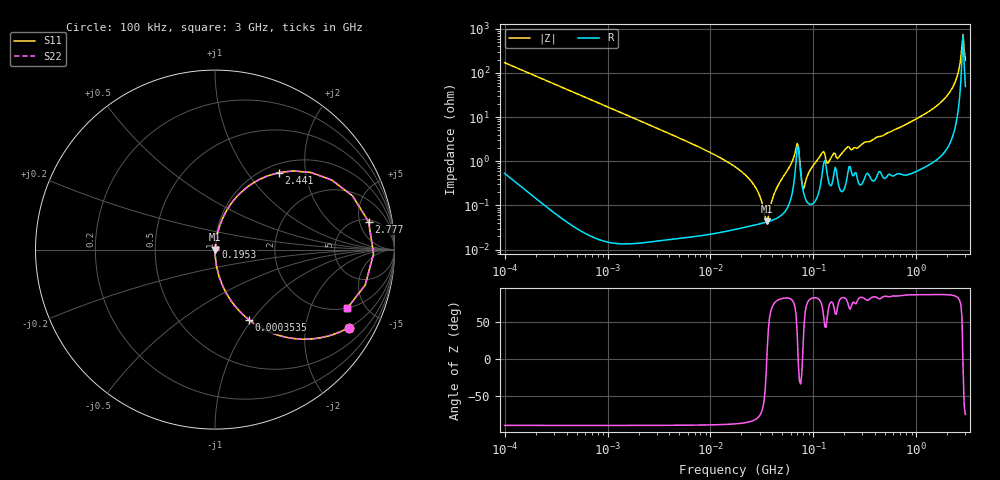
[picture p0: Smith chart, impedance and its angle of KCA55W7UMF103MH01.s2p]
!Murata Part Number: KCA55W7UMF103MH01
!These Parameters are Measured in Series Mode Connection
!Data Generated on Jan 08, 2026
!  o--ll--o
!Port1  Port2
!  o------o
!Operation Temp=25[degC], DC Bias Voltage=0[V]
!Freq. Start=100[kHz] Stop=3[GHz] 401[Steps]
# Hz S RI R 50
!Freq.(Hz) S11(Real) S11(Imag) S21(Real) S21(Imag) S12(Real) S12(Imag) S22(Real) S22(Imag)
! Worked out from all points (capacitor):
!   401 points, 100 kHz to 3 GHz, reference 50 ohm
!   read as one part in series: C = 9.31 nF near 105.3 kHz
!   lowest |Z| = 43.8 mohm at 35.64 MHz (marker M1)
!   series resonance near 35.29 MHz, so ESL is about 2.2 nH
!   S11 on the Smith chart (normalised r, x): 100 kHz: 1.01, -3.42; 353.5 kHz: 1.00, -0.97; 195.3 MHz: 1.00, +0.03; 2.441 GHz: 1.15, +1.43; 2.777 GHz: 5.40, +6.90; 3 GHz: 1.98, -3.71
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100000  0.7442 -0.4348  0.2558 0.4348  0.2558 0.4348  0.7442 -0.4348
353547  0.1898 -0.3916  0.8102 0.3916  0.8102 0.3916  0.1898 -0.3916
562235  0.0848 -0.2782  0.9152 0.2782  0.9152 0.2782  0.0848 -0.2782
3161081  0.00302 -0.0534  0.997 0.0534  0.997 0.0534  0.00302 -0.0534
1.77727e7  0.000342 -0.00722  0.9997 0.00722  0.9997 0.00722  0.000342 -0.00722
2.684345e7  0.000367 -0.00275  0.9996 0.00275  0.9996 0.00275  0.000367 -0.00275
3.564176e7  0.000425 0.000102  0.9996 -0.000102  0.9996 -0.000102  0.000425 0.000102
4.268829e7  0.0005 0.00206  0.9995 -0.00206  0.9995 -0.00206  0.0005 0.00206
6.788584e7  0.0101 0.0164  0.9899 -0.0164  0.9899 -0.0164  0.0101 0.0164
7.147675e7  0.0212 -0.00267  0.9788 0.00267  0.9788 0.00267  0.0212 -0.00267
7.722238e7  0.0032 -0.00119  0.9968 0.00119  0.9968 0.00119  0.0032 -0.00119
8.130716e7  0.00174 0.00187  0.9983 -0.00187  0.9983 -0.00187  0.00174 0.00187
9.738194e7  0.00113 0.00737  0.9989 -0.00737  0.9989 -0.00737  0.00113 0.00737
1.228043e8  0.00624 0.0147  0.9938 -0.0147  0.9938 -0.0147  0.00624 0.0147
1.39694e8  0.00374 0.0085  0.9963 -0.0085  0.9963 -0.0085  0.00374 0.0085
1.952919e8  0.00242 0.0163  0.9976 -0.0163  0.9976 -0.0163  0.00242 0.0163
5.475153e8  0.00713 0.0447  0.9929 -0.0447  0.9929 -0.0447  0.00713 0.0447
1.7917e9  0.0631 0.2147  0.9369 -0.2147  0.9369 -0.2147  0.0631 0.2147
2.441062e9  0.3548 0.4289  0.6452 -0.4289  0.6452 -0.4289  0.3548 0.4289
2.637286e9  0.6499 0.3881  0.3501 -0.3881  0.3501 -0.3881  0.6499 0.3881
2.776789e9  0.8556 0.1558  0.1444 -0.1558  0.1444 -0.1558  0.8556 0.1558
3e9  0.7363 -0.3273  0.2637 0.3273  0.2637 0.3273  0.7363 -0.3273
